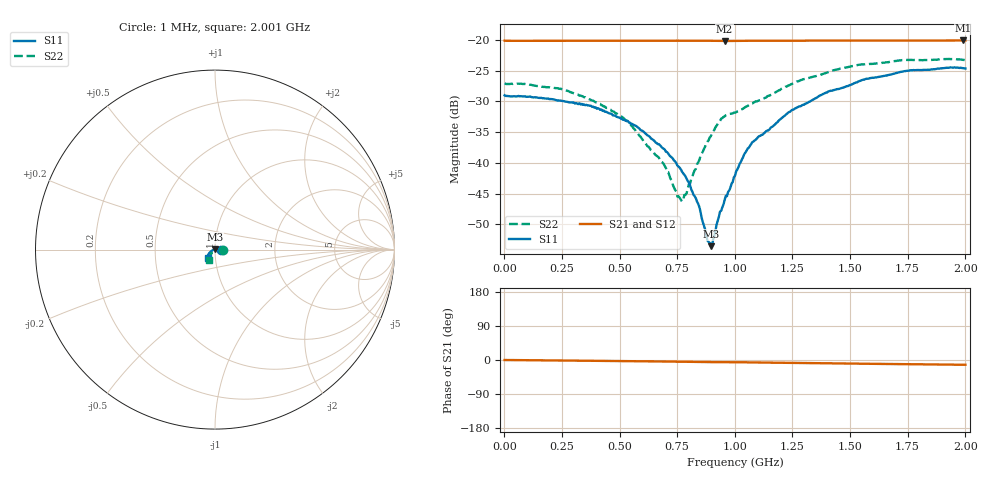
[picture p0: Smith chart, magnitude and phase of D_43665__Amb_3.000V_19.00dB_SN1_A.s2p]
! device id: 43665_
! dir: \\malibu\benchdata\1_engineers\tn_data\43665_75ohm\new\sparar\43665_\amb\3p000v\19p00db
! Serial: 1
! Insertion: A
! Temp: Amb
! VDD: 3.000V
! Attenuation Step: 19.00dB
! IDD: 1.454141e+00mA
! FILE NAME
! DATE 03-27-2009 08:38:00
! CORRECTED  DATA
#  Hz  S  RI  R  75
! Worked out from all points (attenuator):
!   401 points, 1 MHz to 2.001 GHz, reference 75 ohm
!   highest |S21| = -20.07 dB at 1.991 GHz (marker M1); lowest = -20.2 dB at 956 MHz (marker M2)
!   lowest |S11| = -53.5 dB at 896 MHz (marker M3), VSWR 1.00, Z = 74.8 + j0.246 ohm
!   |S11| at or under -10 dB: start of sweep to end of sweep
!   |S22| runs from -46.3 to -23.1 dB; largest |S21 - S12| = 0.00042
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1000000  0.0355 -0.000273  0.0988 -0.000128  0.0988 -0.000207  0.0445 -0.000367
2.36e8  0.032 0.00412  0.0986 -0.00219  0.0986 -0.00215  0.0398 0.00569
3.36e8  0.0298 0.00497  0.0986 -0.00318  0.0986 -0.00315  0.0343 0.00711
5.21e8  0.0214 0.00651  0.0986 -0.00512  0.0986 -0.00503  0.0224 0.00466
6.71e8  0.013 0.00571  0.0985 -0.00658  0.0985 -0.00645  0.011 0.000106
7.01e8  0.0112 0.00528  0.0985 -0.00694  0.0985 -0.00681  0.00908 -0.000769
7.51e8  0.00833 0.0046  0.0985 -0.00756  0.0985 -0.0074  0.00467 -0.00255
7.71e8  0.00719 0.00452  0.0985 -0.00782  0.0985 -0.00762  0.00291 -0.0039
8.36e8  0.00334 0.00354  0.0984 -0.00864  0.0985 -0.00851  -0.00196 -0.00955
8.76e8  0.000199 0.00263  0.0982 -0.00922  0.0983 -0.00903  -0.00489 -0.0135
8.96e8  -0.00132 0.00164  0.0982 -0.00946  0.0982 -0.00926  -0.00668 -0.0151
9.06e8  -0.00208 0.00118  0.0981 -0.00957  0.0982 -0.0094  -0.00798 -0.0161
9.56e8  -0.00497 -0.000377  0.0977 -0.00986  0.0978 -0.00963  -0.0157 -0.0181
1.001e9  -0.00785 -0.00075  0.0979 -0.01  0.098 -0.0098  -0.019 -0.0174
1.046e9  -0.0119 -0.00236  0.0981 -0.0106  0.0983 -0.0104  -0.02 -0.0203
1.081e9  -0.0144 -0.00418  0.0982 -0.0112  0.0983 -0.011  -0.0209 -0.0229
1.241e9  -0.0238 -0.0109  0.0979 -0.0131  0.0981 -0.0129  -0.0261 -0.0345
1.336e9  -0.0284 -0.0158  0.0979 -0.0141  0.0981 -0.0139  -0.0294 -0.0406
1.556e9  -0.0379 -0.0287  0.0975 -0.0168  0.0979 -0.0167  -0.0333 -0.0537
1.671e9  -0.0396 -0.0338  0.0973 -0.0182  0.0975 -0.0181  -0.0343 -0.0568
1.991e9  -0.0378 -0.0453  0.0968 -0.0215  0.0969 -0.0217  -0.0329 -0.0607
2.001e9  -0.0376 -0.0451  0.0968 -0.0216  0.0968 -0.0218  -0.0329 -0.0602
